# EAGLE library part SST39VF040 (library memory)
4 Mbit x8 Multi-Purpose Flash Source: http://www.sst.com/dotAsset/40782.pdf
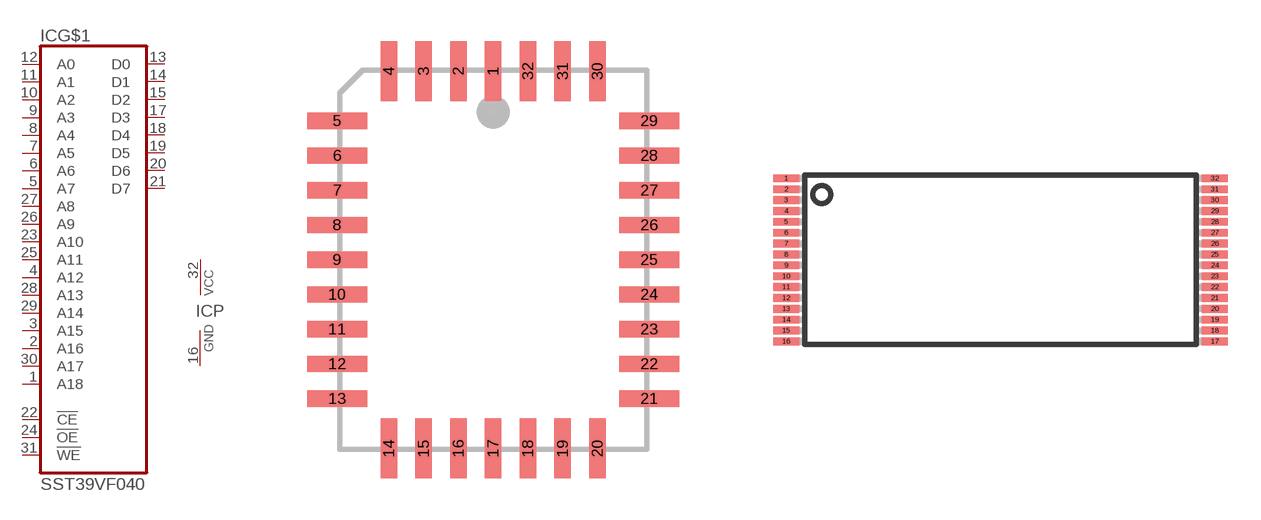
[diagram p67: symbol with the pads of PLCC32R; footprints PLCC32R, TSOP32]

Designator prefix IC; gates G$1=SST39VF040 P=PWRN

## SST39VF040N  [PLCC32R]
1  G$1:A18  in
2  G$1:A16  in
3  G$1:A15  in
4  G$1:A12  in
5  G$1:A7  in
6  G$1:A6  in
7  G$1:A5  in
8  G$1:A4  in
9  G$1:A3  in
10  G$1:A2  in
11  G$1:A1  in
12  G$1:A0  in
13  G$1:D0
14  G$1:D1
15  G$1:D2
16  P:GND  pwr
17  G$1:D3
18  G$1:D4
19  G$1:D5
20  G$1:D6
21  G$1:D7
22  G$1:!CE  in
23  G$1:A10  in
24  G$1:!OE  in
25  G$1:A11  in
26  G$1:A9  in
27  G$1:A8  in
28  G$1:A13  in
29  G$1:A14  in
30  G$1:A17  in
31  G$1:!WE  in
32  P:VCC  pwr

## SST39VF040W  [TSOP32]
1  G$1:A11  in
2  G$1:A9  in
3  G$1:A8  in
4  G$1:A13  in
5  G$1:A14  in
6  G$1:A17  in
7  G$1:!WE  in
8  P:VCC  pwr
9  G$1:A18  in
10  G$1:A16  in
11  G$1:A15  in
12  G$1:A12  in
13  G$1:A7  in
14  G$1:A6  in
15  G$1:A5  in
16  G$1:A4  in
17  G$1:A3  in
18  G$1:A2  in
19  G$1:A1  in
20  G$1:A0  in
21  G$1:D0
22  G$1:D1
23  G$1:D2
24  P:GND  pwr
25  G$1:D3
26  G$1:D4
27  G$1:D5
28  G$1:D6
29  G$1:D7
30  G$1:!CE  in
31  G$1:A10  in
32  G$1:!OE  in

## Footprint PLCC32R (pad centres in mm)
PLASTIC LEADED CHIP CARRIER rectangle
smd 0.6 x 2.2: 1 0,6.9; 2 -1.27,6.9; 3 -2.54,6.9; 4 -3.81,6.9; 14 -3.81,-6.9; 15 -2.54,-6.9; 16 -1.27,-6.9; 17 0,-6.9; 18 1.27,-6.9; 19 2.54,-6.9; 20 3.81,-6.9; 30 3.81,6.9; 31 2.54,6.9; 32 1.27,6.9
smd 2.2 x 0.6: 5 -5.7,5.08; 6 -5.7,3.81; 7 -5.7,2.54; 8 -5.7,1.27; 9 -5.7,0; 10 -5.7,-1.27; 11 -5.7,-2.54; 12 -5.7,-3.81; 13 -5.7,-5.08; 21 5.7,-5.08; 22 5.7,-3.81; 23 5.7,-2.54; 24 5.7,-1.27; 25 5.7,0; 26 5.7,1.27; 27 5.7,2.54; 28 5.7,3.81; 29 5.7,5.08

## Footprint TSOP32 (pad centres in mm)
Thin Small Outline Package
smd 1.2 x 0.36: 1 -9.85,3.75; 2 -9.85,3.25; 3 -9.85,2.75; 4 -9.85,2.25; 5 -9.85,1.75; 6 -9.85,1.25; 7 -9.85,0.75; 8 -9.85,0.25; 9 -9.85,-0.25; 10 -9.85,-0.75; 11 -9.85,-1.25; 12 -9.85,-1.75; 13 -9.85,-2.25; 14 -9.85,-2.75; 15 -9.85,-3.25; 16 -9.85,-3.75; 17 9.85,-3.75; 18 9.85,-3.25; 19 9.85,-2.75; 20 9.85,-2.25; 21 9.85,-1.75; 22 9.85,-1.25; 23 9.85,-0.75; 24 9.85,-0.25; 25 9.85,0.25; 26 9.85,0.75; 27 9.85,1.25; 28 9.85,1.75; 29 9.85,2.25; 30 9.85,2.75; 31 9.85,3.25; 32 9.85,3.75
